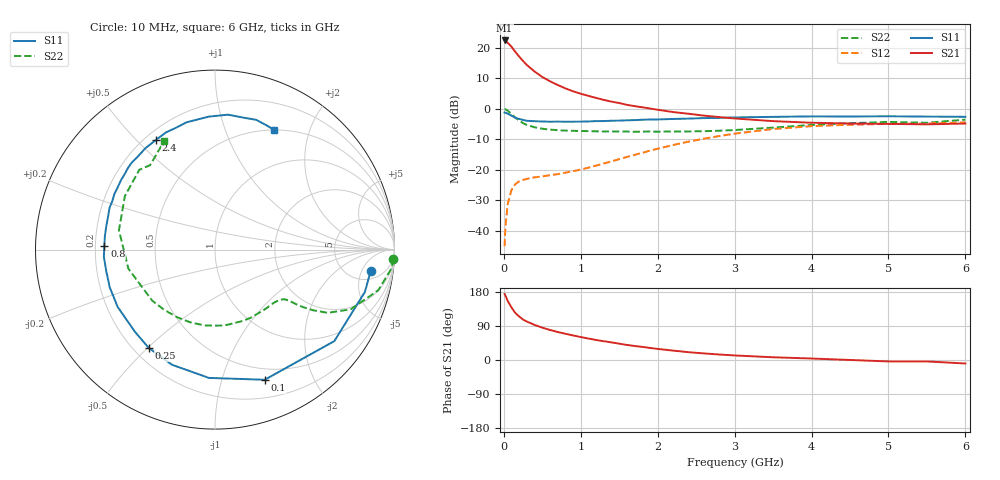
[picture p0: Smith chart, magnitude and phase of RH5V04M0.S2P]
! SIEMENS Small Signal Semiconductors
! BFR106
! Si NPN RF Bipolar Junction Transistor in SOT23
! VCE = 5 V  IC = 4 mA
! Common Emitter S-Parameters:  August  1996
# GHz  S  MA  R  50
!  f  S11  S21  S12  S22
! GHz  MAG  ANG  MAG  ANG  MAG  ANG  MAG  ANG
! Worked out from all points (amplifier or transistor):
!   36 points, 10 MHz to 6 GHz, reference 50 ohm
!   highest |S21| = 22.5 dB at 10 MHz (marker M1)
!   |S21| within 3 dB of that: start of sweep to 127.2 MHz
!   unconditionally stable (mu >= 1): 675.6 MHz to 1.845 GHz; 4.585 GHz to end of sweep
!   at 250 MHz: K = 0.45, MSG = 19.5 dB, |S12| = -23.3 dB
!   at 1.4 GHz: K = 1.16, MAG = 7.4 dB, |S12| = -17.2 dB
!   at 6 GHz: K = 1.02, MAG = -1.1 dB, |S12| = -4.4 dB
!   S11 on the Smith chart (normalised r, x): 10 MHz: 7, -7; 100 MHz: 0.38, -1.38; 250 MHz: 0.26, -0.50; 800 MHz: 0.24, +0.01; 2.4 GHz: 0.24, +0.57; 6 GHz: 0.50, +1.49
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0.01  0.8754 -7.9  13.31 174.3  0.0056 86.8  0.9949 -3.0
0.02  0.8678 -15.8  13.14 170.3  0.0114 80.8  0.9898 -6.0
0.05  0.8378 -37.5  12.22 156.1  0.0275 70.5  0.9373 -14.0
0.1  0.7762 -69.1  10.49 138.3  0.0469 56.5  0.8254 -23.8
0.15  0.7157 -92.7  8.614 123.9  0.0585 47.1  0.72 -29.3
0.2  0.6849 -110.5  7.225 114.7  0.065 41.7  0.6437 -31.7
0.25  0.6603 -124.0  6.114 106.7  0.0687 38.4  0.5845 -33.2
0.3  0.6396 -134.1  5.258 101.4  0.0714 37.3  0.5477 -33.9
0.4  0.6293 -149.5  4.111 92.6  0.0755 36.6  0.4998 -34.6
0.5  0.6229 -160.3  3.348 85.3  0.078 37.7  0.4733 -35.7
0.6  0.6176 -169.0  2.844 79.3  0.0819 40.1  0.4582 -37.6
0.8  0.6169 178.3  2.177 69.2  0.0899 46.5  0.4413 -42.4
0.9  0.6181 173.0  1.949 64.8  0.0953 50.0  0.4374 -44.9
1.1  0.6236 162.8  1.638 56.6  0.1089 56.0  0.4322 -51.6
1.6  0.6509 143.7  1.168 39.8  0.1628 64.7  0.425 -70.5
2.2  0.685 124.5  0.89 24.8  0.2558 63.0  0.4264 -97.9
2.4  0.6943 118.2  0.835 20.6  0.2908 60.6  0.428 -108.9
3.5  0.7417 92.7  0.631 7.2  0.4691 39.9  0.4941 -167.5
4.5  0.7521 77.8  0.577 0.1  0.5518 19.1  0.5839 149.3
5  0.7585 72.4  0.569 -3.8  0.5688 10.8  0.6128 133.5
5.5  0.7492 67.2  0.559 -3.8  0.5759 6.5  0.5934 127.5
6  0.7432 63.6  0.577 -9.2  0.6034 -1.6  0.6668 115.2
